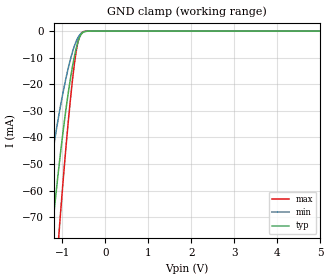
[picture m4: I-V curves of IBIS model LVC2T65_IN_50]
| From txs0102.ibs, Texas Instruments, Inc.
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[Model]   LVC2T65_IN_50
Model_type  Input
Vinl=1.575
Vinh=3.575
| variable   typ   min   max
C_comp   2.79pF   2.38pF   3.25pF
[Temperature Range]   40   100   -40
| Ambient temperature   25   85   -40
[Voltage range]   5   4.5   5.5
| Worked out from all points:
|   GND clamp passes 1 mA (typ) near -0.55 V on its own axis
[GND Clamp]
| LVC2T65_IN_50
|   Voltage   I(typ)   I(min)   I(max)
-5.5V     -1.044A    -791.8mA   -1.306A
-1.485V   -117.8mA   -75.58mA   -171.6mA
-1.235V   -74.52mA   -46.69mA   -110.8mA
-1.095V   -53.01mA   -32.74mA   -79.35mA
-1.07V    -49.42mA   -30.43mA   -74mA
-890mV    -26.16mA   -15.73mA   -38.65mA
-815mV    -18.03mA   -10.7mA    -25.91mA
-735mV    -10.64mA   -6.252mA   -14.08mA
-675mV    -6.184mA   -3.665mA   -7.196mA
-625mV    -3.366mA   -2.081mA   -3.292mA
-520mV    -498.4uA   -390.9uA   -269.3uA
5V        315.4pA    1.086nA    37.11pA
